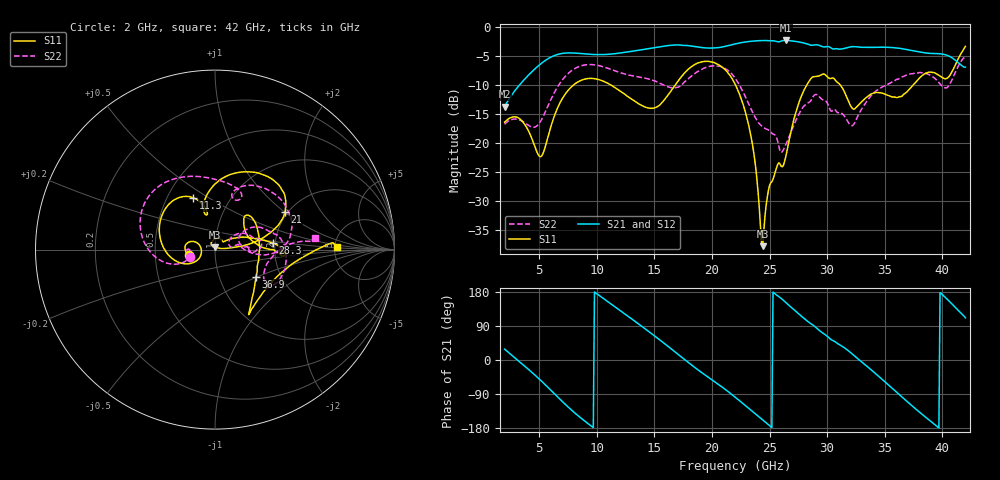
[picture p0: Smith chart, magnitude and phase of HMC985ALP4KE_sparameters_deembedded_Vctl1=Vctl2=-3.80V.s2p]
!s2p File: Measurements: S11, S21, S12, S22
# GHz S dB R 50.0
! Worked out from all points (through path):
!   401 points, 2 GHz to 42 GHz, reference 50 ohm
!   highest |S21| = -2.31 dB at 26.4 GHz (marker M1); lowest = -13.8 dB at 2 GHz (marker M2)
!   lowest |S11| = -37.8 dB at 24.4 GHz (marker M3), VSWR 1.03, Z = 50 + j1.28 ohm
!   |S11| at or under -10 dB: start of sweep to 7.983 GHz; 22.04 GHz to 28.24 GHz (6.192 GHz wide, 24.6 % of centre); 31.13 GHz to 37.46 GHz (6.322 GHz wide, 18.4 % of centre)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
!   |S22| runs from -21.7 to -5.0 dB; largest |S21 - S12| = 0.00068
!   S11 on the Smith chart (normalised r, x): 2 GHz: 0.74, -0.05; 11.3 GHz: 0.67, +0.43; 21 GHz: 1.94, +1.00; 28.3 GHz: 1.94, +0.16; 36.9 GHz: 1.50, -0.49; 42 GHz: 5.24, +0.31
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2  -16.44 -168.2  -13.76 28.6  -13.76 28.6  -16.79 -163.0
3.4  -16.00 166.7  -9.75 -7.4  -9.76 -7.4  -16.14 179.9
5.2  -22.32 -170.1  -6.25 -55.7  -6.25 -55.7  -16.01 -161.2
6.8  -13.11 -162.3  -4.63 -103.4  -4.63 -103.4  -9.72 -171.6
8.7  -9.15 149.5  -4.59 -155.0  -4.59 -155.0  -6.66 150.5
11.3  -10.10 112.6  -4.65 146.5  -4.66 146.5  -7.35 107.8
13.5  -13.06 102.3  -4.04 98.0  -4.04 98.0  -8.58 76.9
15.4  -13.57 106.0  -3.43 54.7  -3.43 54.7  -9.64 63.2
17.9  -7.36 78.1  -3.20 -5.4  -3.20 -5.4  -8.99 70.9
21  -7.11 28.1  -3.40 -74.1  -3.40 -74.1  -6.98 16.7
22  -9.81 17.0  -2.92 -97.7  -2.92 -97.7  -8.80 0.0
23.4  -19.02 6.7  -2.45 -132.6  -2.45 -132.6  -14.20 -4.4
24.4  -37.85 87.5  -2.33 -157.9  -2.33 -157.8  -17.26 9.4
25  -27.35 120.4  -2.36 -173.2  -2.36 -173.2  -17.90 12.5
26.4  -22.45 40.0  -2.31 152.0  -2.31 152.0  -20.33 33.5
28.3  -9.78 6.6  -2.94 102.1  -2.94 102.1  -13.14 18.2
28.7  -8.67 0.5  -3.14 93.7  -3.15 93.6  -12.31 15.4
32.4  -14.13 31.0  -3.39 10.0  -3.39 10.0  -16.49 26.9
35.4  -11.88 15.7  -3.51 -68.0  -3.50 -68.0  -9.76 17.6
36.9  -11.24 -33.4  -3.88 -108.5  -3.88 -108.5  -8.28 4.4
39.7  -8.33 -56.2  -4.60 -179.4  -4.60 -179.4  -9.61 -33.3
42  -3.35 1.3  -6.92 111.1  -6.92 111.1  -5.04 6.6
